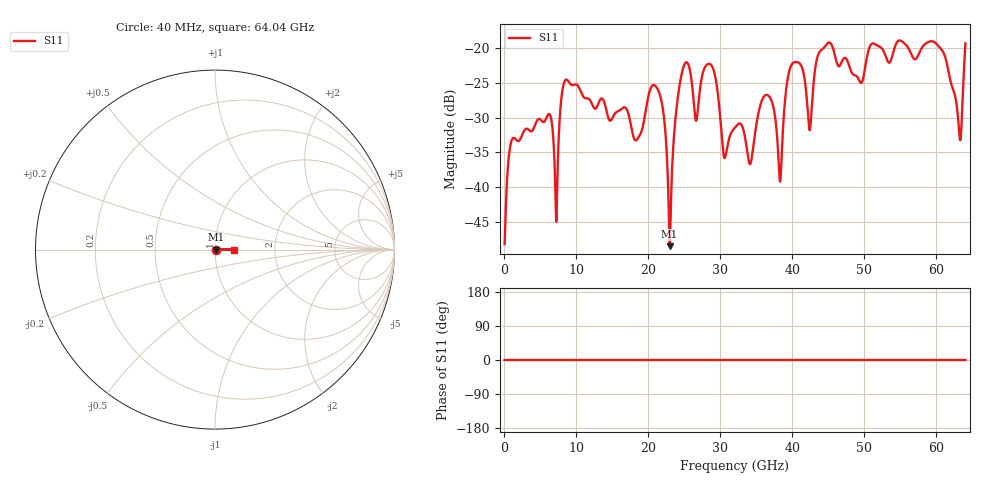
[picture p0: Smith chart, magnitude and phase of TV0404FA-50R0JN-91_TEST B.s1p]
! FILE NAME
! DATE 02/23/2016  13:53
! CORRECTED  DATA
# GHz  S  DB  R  50
!  FREQ  S11M  S11A
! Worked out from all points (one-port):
!   1601 points, 40 MHz to 64.04 GHz, reference 50 ohm
!   lowest |S11| = -48.5 dB at 22.96 GHz (marker M1), VSWR 1.01, Z = 50.4 + j0 ohm
!   |S11| at or under -10 dB: start of sweep to end of sweep
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0.04  -48.21 0.0
1.24  -32.93 0.0
6.24  -29.48 0.0
7.24  -44.80 0.0
8.08  -25.98 0.0
16.08  -28.92 0.0
18.4  -33.18 0.0
21.28  -25.86 0.0
22.2  -30.21 0.0
22.96  -48.51 0.0
24.08  -27.25 0.0
25.36  -22.04 0.0
26.68  -30.41 0.0
28.56  -22.28 0.0
30.56  -35.81 0.0
32.08  -31.37 0.0
34.16  -36.68 0.0
36.68  -26.83 0.0
38.28  -39.17 0.0
40.08  -22.14 0.0
41.4  -22.92 0.0
42.4  -31.80 0.0
43.96  -20.32 0.0
48.08  -23.07 0.0
56.08  -19.92 0.0
60.8  -20.30 0.0
63.24  -32.79 0.0
64.04  -19.30 0.0
